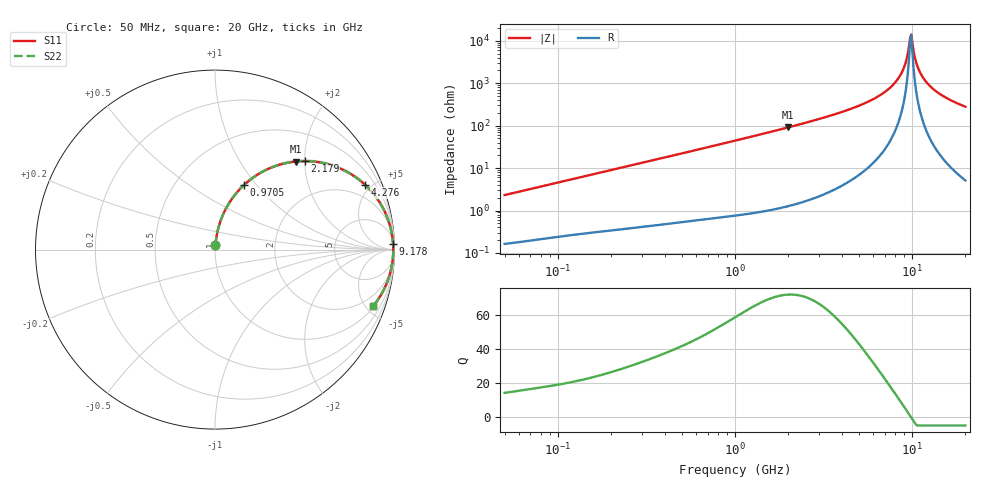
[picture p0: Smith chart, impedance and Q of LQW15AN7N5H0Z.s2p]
!Murata Part Number: LQW15AN7N5H0Z
!These Parameters are Measured in Series Mode Connection
!  o--[Z]--o
!Port1  Port2
!  o-------o
!Freq. Start=50[MHz] Stop=20[GHz], 401[Steps]
# Hz S RI R 50
!Freq.(Hz) S11(Real) S11(Imag) S21(Real) S21(Imag) S12(Real) S12(Imag) S22(Real) S22(Imag)
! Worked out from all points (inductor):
!   401 points, 50 MHz to 20 GHz, reference 50 ohm
!   read as one part in series: L = 7.3 nH near 51.52 MHz
!   highest Q = 71.9 at 1.992 GHz (marker M1), where L = 7.25 nH
!   self-resonance near 9.745 GHz
!   S11 on the Smith chart (normalised r, x): 50 MHz: 1.00, +0.05; 970.5 MHz: 1.01, +0.86; 2.179 GHz: 1.03, +2.00; 4.276 GHz: 1.09, +4.60; 9.178 GHz: 13, +58; 20 GHz: 1.10, -5.59
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5e7  0.00216 0.023  0.9978 -0.023  0.9978 -0.023  0.00216 0.023
1.364002e8  0.00654 0.0609  0.9935 -0.0609  0.9935 -0.0609  0.00654 0.0609
3.721004e8  0.0306 0.159  0.9694 -0.159  0.9694 -0.159  0.0306 0.159
9.70487e8  0.1599 0.3579  0.8401 -0.3579  0.8401 -0.3579  0.1599 0.3579
1e9  0.168 0.3654  0.832 -0.3654  0.832 -0.3654  0.168 0.3654
1.99176e9  0.452 0.4908  0.548 -0.4908  0.548 -0.4908  0.452 0.4908
2.179053e9  0.5002 0.4931  0.4998 -0.4931  0.4998 -0.4931  0.5002 0.4931
2.728004e9  0.6228 0.4775  0.3772 -0.4775  0.3772 -0.4775  0.6228 0.4775
4.275624e9  0.8361 0.3606  0.1639 -0.3606  0.1639 -0.3606  0.8361 0.3606
5.944466e9  0.9371 0.228  0.0629 -0.228  0.0629 -0.228  0.9371 0.228
7.442007e9  0.9761 0.1281  0.0239 -0.1281  0.0239 -0.1281  0.9761 0.1281
8.516016e9  0.9886 0.0667  0.0114 -0.0667  0.0114 -0.0667  0.9886 0.0667
9.178299e9  0.9921 0.0324  0.0079 -0.0324  0.0079 -0.0324  0.9921 0.0324
9.600142e9  0.9931 0.0118  0.00694 -0.0118  0.00694 -0.0118  0.9931 0.0118
9.892087e9  0.9932 -0.00194  0.00678 0.00194  0.00678 0.00194  0.9932 -0.00194
1.004137e10  0.9932 -0.00882  0.00685 0.00882  0.00685 0.00882  0.9932 -0.00882
1.050288e10  0.9924 -0.0294  0.00761 0.0294  0.00761 0.0294  0.9924 -0.0294
1.082228e10  0.9914 -0.0432  0.0086 0.0432  0.0086 0.0432  0.9914 -0.0432
1.131968e10  0.9892 -0.0638  0.0108 0.0638  0.0108 0.0638  0.9892 -0.0638
1.220001e10  0.9836 -0.098  0.0164 0.098  0.0164 0.098  0.9836 -0.098
1.504638e10  0.9546 -0.1926  0.0454 0.1926  0.0454 0.1926  0.9546 -0.1926
2e10  0.882 -0.3136  0.118 0.3136  0.118 0.3136  0.882 -0.3136
